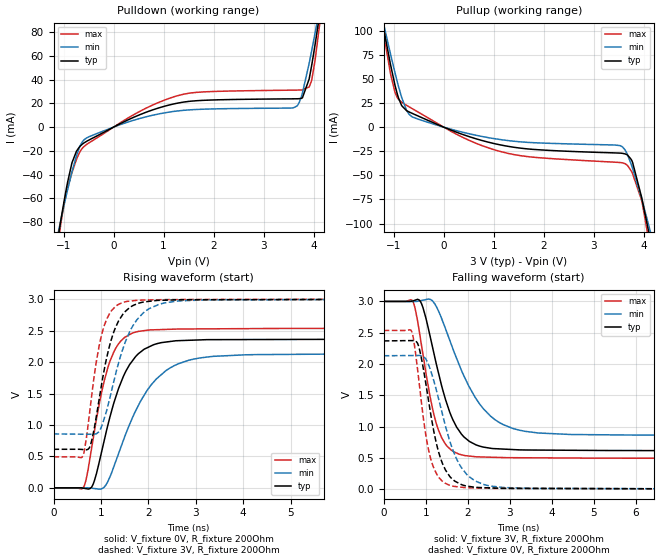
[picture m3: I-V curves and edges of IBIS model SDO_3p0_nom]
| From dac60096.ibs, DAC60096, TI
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|   Model
[Model]   SDO_3p0_nom
Model_type   Output
Polarity   Non-Inverting
Vmeas = 1.5
Vref = 0
Cref = 1pF
Rref = 100000
|   typ   min   max
C_comp   13.124pF   12.937pF   13.913pF
[Voltage Range]   3   2.999   3.001
[Temperature Range]   27   105   -40
[Pullup Reference]   3   2.999   3.001
[Pulldown Reference]   0   0   0
[Power Clamp Reference]   3   2.999   3.001
[GND Clamp Reference]   0   0   0
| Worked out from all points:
|   slope of the pulldown table from 0 to 0.45 V, typ, clamps not added: 49.3 ohm
|   slope of the pullup table from 0 to 0.45 V, typ, clamps not added: 51 ohm
|   falling waveform, V_fixture 3V, R_fixture 200Ohm: 20-80 % time 582ps typ, 902ps min, 425ps max; typ from 3 V to 0.614 V
|   rising waveform, V_fixture 0V, R_fixture 200Ohm: 20-80 % time 572ps typ, 823ps min, 422ps max; typ from 0 V to 2.37 V
|   rising waveform, V_fixture 3V, R_fixture 200Ohm: 20-80 % time 401ps typ, 530ps min, 310ps max; typ from 0.613 V to 3 V
|   falling waveform, V_fixture 0V, R_fixture 200Ohm: 20-80 % time 412ps typ, 573ps min, 325ps max; typ from 2.37 V to 0 V
[Pulldown]
|   Voltage   I(typ)   I(min)   I(max)
-3V       -641.5mA   -522.3mA   -768.1mA
-1.173V   -109.3mA   -102mA     -118.2mA
-1.047V   -76.61mA   -76.83mA   -79.26mA
-831mV    -29.98mA   -37.56mA   -38.24mA
-633mV    -14.65mA   -12.99mA   -18.28mA
114mV     2.513mA    1.781mA    3.141mA
1.401V    21.09mA    14.15mA    27.74mA
3.669V    23.88mA    17.79mA    31.2mA
3.777V    24.68mA    28.68mA    31.38mA
3.957V    50.68mA    63.17mA    38.62mA
4.137V    98.94mA    103.4mA    91.47mA
6V        669.1mA    557.5mA    817.1mA
[Pullup]
|   Voltage   I(typ)   I(min)   I(max)
-3V       652.6mA    545.1mA    798.5mA
-1.263V   120.3mA    121.2mA    120.7mA
-1.182V   97.06mA    102.4mA    91.95mA
-1.065V   65.14mA    75.98mA    55.44mA
-930mV    34.59mA    47.28mA    30.65mA
-741mV    17.02mA    17.18mA    22.54mA
-489mV    11.01mA    7.889mA    14.95mA
1.149V    -18.59mA   -13mA      -25.47mA
3.561V    -27.09mA   -19.98mA   -36.92mA
3.777V    -36.6mA    -42.72mA   -48.2mA
4.101V    -109mA     -102.1mA   -117.3mA
6V        -661.7mA   -537.8mA   -793.8mA
[Ramp]
R_load = 200
|   typ   min   max
dV/dt_r   1.42112/5.7093e-10   1.2785/8.20147e-10   1.52161/4.20742e-10
dV/dt_f   1.43185/5.81046e-10   1.28409/9.02e-10   1.50481/4.25021e-10
[Falling Waveform]
V_fixture = 3V
V_fixture_min = 2.999V
V_fixture_max = 3.001V
R_fixture = 200Ohm
C_fixture = 0F
|   Time   V(typ)   V(min)   V(max)
0s        3V         2.999V     3.001V
671.2ps   3.004V     2.999V     3.018V
873.5ps   2.999V     3.012V     2.406V
1.096ns   2.463V     3.033V     1.502V
1.275ns   1.933V     2.885V     996.9mV
1.567ns   1.235V     2.385V     648.2mV
1.789ns   938mV      1.998V     560.6mV
2.368ns   672.6mV    1.286V     513.8mV
3.211ns   628.5mV    944.7mV    502.4mV
10ns      613.6mV    858.9mV    493mV
[Rising Waveform]
V_fixture = 0V
V_fixture_min = 0V
V_fixture_max = 0V
R_fixture = 200Ohm
C_fixture = 0F
|   Time   V(typ)   V(min)   V(max)
0s        -64.52nV   -330.1nV   -13.69nV
615.4ps   -3.426mV   617uV      -6.284mV
808.5ps   17.76mV    -5.527mV   654mV
1.009ns   556mV      -15.4mV    1.499V
1.195ns   1.142V     183.8mV    2.024V
1.47ns    1.766V     749.3mV    2.37V
1.657ns   2.012V     1.101V     2.458V
2.171ns   2.289V     1.733V     2.514V
3.08ns    2.352V     2.065V     2.527V
10ns      2.369V     2.131V     2.536V
[Rising Waveform]
V_fixture = 3V
V_fixture_min = 2.999V
V_fixture_max = 3.001V
R_fixture = 200Ohm
C_fixture = 0F
|   Time   V(typ)   V(min)   V(max)
0s        613.2mV    857.3mV    492.9mV
603ps     610.5mV    853.4mV    488.8mV
758.5ps   641.6mV    852.4mV    1.181V
909.6ps   1.167V     863.2mV    2.036V
1.049ns   1.794V     1.054V     2.528V
1.252ns   2.437V     1.629V     2.84V
1.459ns   2.756V     2.201V     2.946V
1.889ns   2.953V     2.779V     2.985V
2.64ns    2.989V     2.971V     2.993V
10ns      3V         2.999V     3.001V
[Falling Waveform]
|Gnd
V_fixture = 0V
V_fixture_min = 0V
V_fixture_max = 0V
R_fixture = 200Ohm
C_fixture = 0F
|   Time   V(typ)   V(min)   V(max)
0s        2.369V     2.132V     2.536V
646.1ps   2.374V     2.135V     2.54V
803.8ps   2.332V     2.136V     1.922V
977.4ps   1.786V     2.098V     968.1mV
1.122ns   1.18V      1.881V     474.3mV
1.308ns   588.7mV    1.436V     190.2mV
1.547ns   226.6mV    820.9mV    67.75mV
1.977ns   48.72mV    233.1mV    23.31mV
2.544ns   20.08mV    49.46mV    13.55mV
10ns      460.1uV    1.303mV    105.4uV
